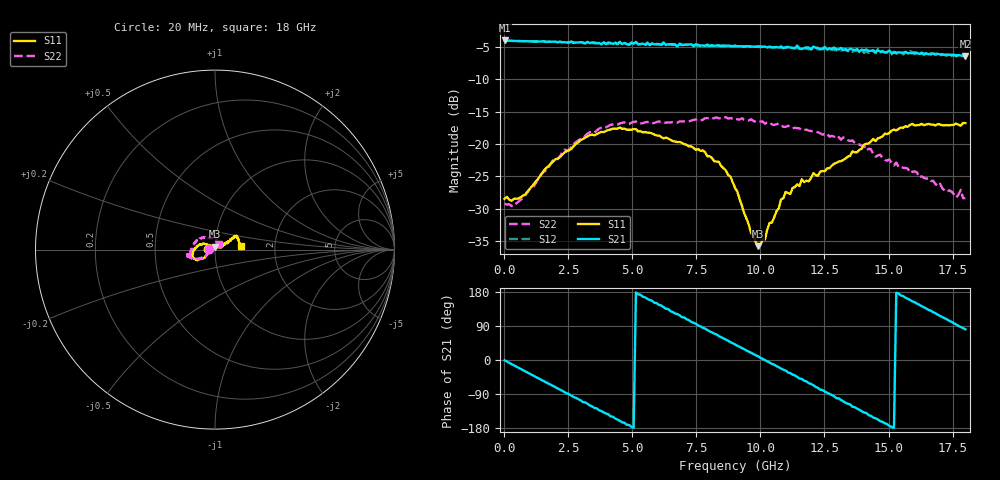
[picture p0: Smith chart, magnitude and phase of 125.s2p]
!Agilent Technologies,N5230A,US43500223,A.07.50.48
!Agilent N5230A: A.07.50.48
!Date: Monday, February 01, 2016 16:37:41
!Correction: S11(Full 2 Port(1,2))
!S21(Full 2 Port(1,2))
!S12(Full 2 Port(1,2))
!S22(Full 2 Port(1,2))
!S2P File: Measurements: S11, S21, S12, S22:
# Hz S  RI  R 50
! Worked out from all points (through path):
!   201 points, 20 MHz to 18 GHz, reference 50 ohm
!   highest |S21| = -3.96 dB at 20 MHz (marker M1); lowest = -6.4 dB at 18 GHz (marker M2)
!   group delay of S21, straight-line fit = 98.4 ps
!   lowest |S11| = -35.8 dB at 9.909 GHz (marker M3), VSWR 1.03, Z = 50.1 + j1.62 ohm
!   |S11| at or under -10 dB: start of sweep to end of sweep
!   |S22| runs from -29.6 to -15.9 dB; largest |S21 - S12| = 0.031
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2e7  -0.0377 0.0014  0.6341 -0.00879  0.6343 -0.0094  -0.0344 0.00067
8.291e8  -0.0366 -0.018  0.5417 -0.3135  0.5409 -0.3148  -0.0364 -0.017
1.5483e9  -0.051 -0.0357  0.351 -0.5164  0.3489 -0.5172  -0.0494 -0.0359
2.1776e9  -0.0637 -0.0469  0.128 -0.6075  0.1248 -0.6054  -0.0685 -0.0421
3.0766e9  -0.0937 -0.0567  -0.2198 -0.5662  -0.217 -0.5715  -0.0987 -0.0507
4.515e9  -0.1275 -0.042  -0.5803 -0.2049  -0.5867 -0.2037  -0.1379 -0.0429
5.1443e9  -0.1278 -0.0251  -0.6156 0.0217  -0.6182 0.0288  -0.1448 -0.0378
6.0433e9  -0.1164 0.000601  -0.4905 0.3398  -0.4778 0.3476  -0.1467 -0.0283
7.4817e9  -0.0859 0.0277  -0.0577 0.5908  -0.0404 0.5808  -0.152 -0.0305
8.3807e9  -0.065 0.0328  0.2634 0.5189  0.2659 0.511  -0.1556 -0.0299
9.01e9  -0.0384 0.025  0.4362 0.3803  0.4373 0.3682  -0.1527 -0.0379
9.909e9  0.00121 0.0161  0.5623 0.0983  0.5599 0.0819  -0.1447 -0.0342
1.01787e10  0.0139 0.0118  0.5692 -0.0039  0.5633 -0.0139  -0.1397 -0.0342
1.09878e10  0.0392 0.0168  0.4971 -0.2644  0.4823 -0.2827  -0.1353 -0.0122
1.20666e10  0.0535 0.026  0.2261 -0.5219  0.1974 -0.5126  -0.1228 0.0256
1.26959e10  0.0559 0.0333  0.00802 -0.5489  -0.0231 -0.5498  -0.1064 0.0411
1.3505e10  0.0719 0.0378  -0.2518 -0.4848  -0.2697 -0.462  -0.0874 0.0595
1.45838e10  0.0932 0.0598  -0.4892 -0.2105  -0.504 -0.2014  -0.0462 0.0674
1.50333e10  0.1013 0.0679  -0.5267 -0.0575  -0.5087 -0.04  -0.0326 0.0687
1.58424e10  0.1181 0.0771  -0.4716 0.1858  -0.4859 0.1946  -0.00954 0.0591
1.67414e10  0.1284 0.0599  -0.2948 0.4047  -0.2796 0.4193  0.00464 0.0517
1.8e10  0.1441 0.0194  0.0751 0.4725  0.1006 0.4682  0.0246 0.0292
